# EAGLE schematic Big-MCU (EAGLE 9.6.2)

## Sheet 1 of 5: Board to Board Headers
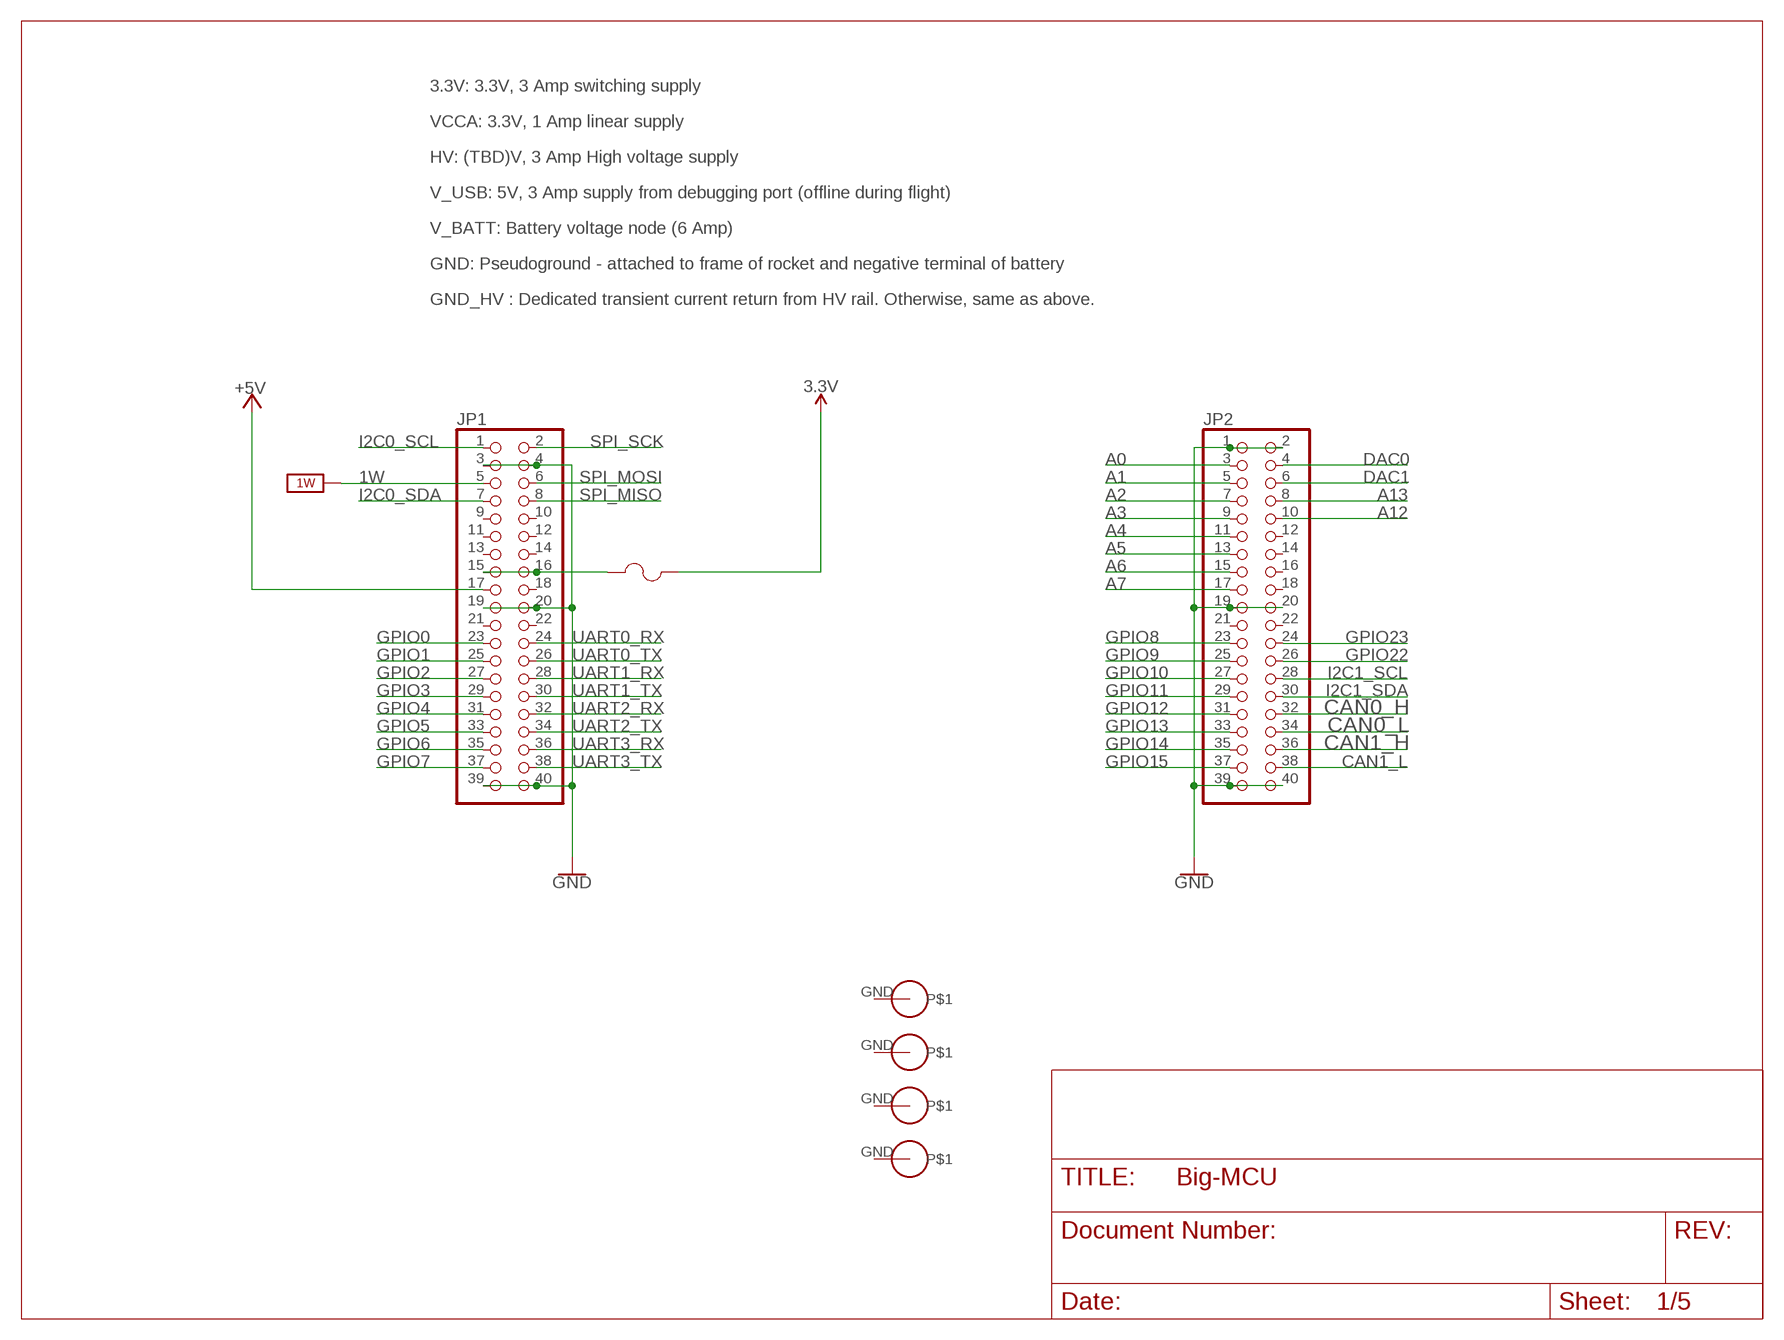
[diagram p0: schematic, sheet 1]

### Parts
$$U$1  PS/104-MOUNTING-HOLE  [PC/104-MOUNTING-HOLE]
F1  0603SFF150F/32-2  [FUS0603_TYCO]
JP1  PINHD-2X20  [2X20]
JP2  PINHD-2X20  [2X20]
U$1  PS/104-MOUNTING-HOLE  [PC/104-MOUNTING-HOLE]
U$2  PS/104-MOUNTING-HOLE  [PC/104-MOUNTING-HOLE]
U$3  PS/104-MOUNTING-HOLE  [PC/104-MOUNTING-HOLE]

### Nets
1W: JP1.5 ; supply symbol labelled 1W_SUP ; also sheet 3
3.3V [New Class]: F1.2 ; also sheet 2,4
+5V: JP1.17 ; also sheet 5
A0: JP2.3 ; also sheet 2
A1: JP2.5 ; also sheet 2
A2: JP2.7 ; also sheet 2
A3: JP2.9 ; also sheet 2
A4: JP2.11 ; also sheet 2
A5: JP2.13 ; also sheet 2
A6: JP2.15 ; also sheet 2
A7: JP2.17 ; also sheet 2
A12: JP2.10 ; also sheet 2
A13: JP2.8 ; also sheet 2
CAN0_H: JP2.32 ; also sheet 5
CAN0_L: JP2.34 ; also sheet 5
CAN1_H: JP2.36 ; also sheet 5
CAN1_L: JP2.38 ; also sheet 5
DAC0: JP2.4 ; also sheet 2
DAC1: JP2.6 ; also sheet 2
GND [New Class]: JP1.3 JP1.4 JP1.19 JP1.20 JP1.39 JP1.40 JP2.1 JP2.2 JP2.19 JP2.20 JP2.39 JP2.40 ; also sheet 2,3,4,5
GPIO0: JP1.23 ; also sheet 2
GPIO1: JP1.25 ; also sheet 2
GPIO2: JP1.27 ; also sheet 2
GPIO3: JP1.29 ; also sheet 2
GPIO4: JP1.31 ; also sheet 2
GPIO5: JP1.33 ; also sheet 2
GPIO6: JP1.35 ; also sheet 2
GPIO7: JP1.37 ; also sheet 2
GPIO8: JP2.23 ; also sheet 2
GPIO9: JP2.25 ; also sheet 2
GPIO10: JP2.27 ; also sheet 2
GPIO11: JP2.29 ; also sheet 2
GPIO12: JP2.31 ; also sheet 2
GPIO13: JP2.33 ; also sheet 2
GPIO14: JP2.35 ; also sheet 2
GPIO15: JP2.37 ; also sheet 2
GPIO22: JP2.26 ; also sheet 2
GPIO23: JP2.24 ; also sheet 2
I2C0_SCL: JP1.1 ; also sheet 2,3
I2C0_SDA: JP1.7 ; also sheet 2,3
I2C1_SCL: JP2.28 ; also sheet 2
I2C1_SDA: JP2.30 ; also sheet 2
N$3: F1.1 JP1.15 JP1.16
SPI_MISO: JP1.8 ; also sheet 2
SPI_MOSI: JP1.6 ; also sheet 4
SPI_SCK: JP1.2 ; also sheet 4
UART0_RX: JP1.24 ; also sheet 2
UART0_TX: JP1.26 ; also sheet 2
UART1_RX: JP1.28 ; also sheet 2
UART1_TX: JP1.30 ; also sheet 2
UART2_RX: JP1.32 ; also sheet 2
UART2_TX: JP1.34 ; also sheet 2
UART3_RX: JP1.36 ; also sheet 2
UART3_TX: JP1.38 ; also sheet 2
Unconnected: $$U$1.GND JP1.9 JP1.10 JP1.11 JP1.12 JP1.13 JP1.14 JP1.18 JP1.21 JP1.22 JP2.12 JP2.14 JP2.16 JP2.18 JP2.21 JP2.22 U$1.GND U$2.GND U$3.GND

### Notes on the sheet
- 3.3V: 3.3V, 3 Amp switching supply
- VCCA: 3.3V, 1 Amp linear supply
- HV: (TBD)V, 3 Amp High voltage supply
- V_USB: 5V, 3 Amp supply from debugging port (offline during flight)
- V_BATT: Battery voltage node (6 Amp)
- GND: Pseudoground - attached to frame of rocket and negative terminal of battery
- GND_HV : Dedicated transient current return from HV rail. Otherwise, same as above.

## Sheet 2 of 5: MCU
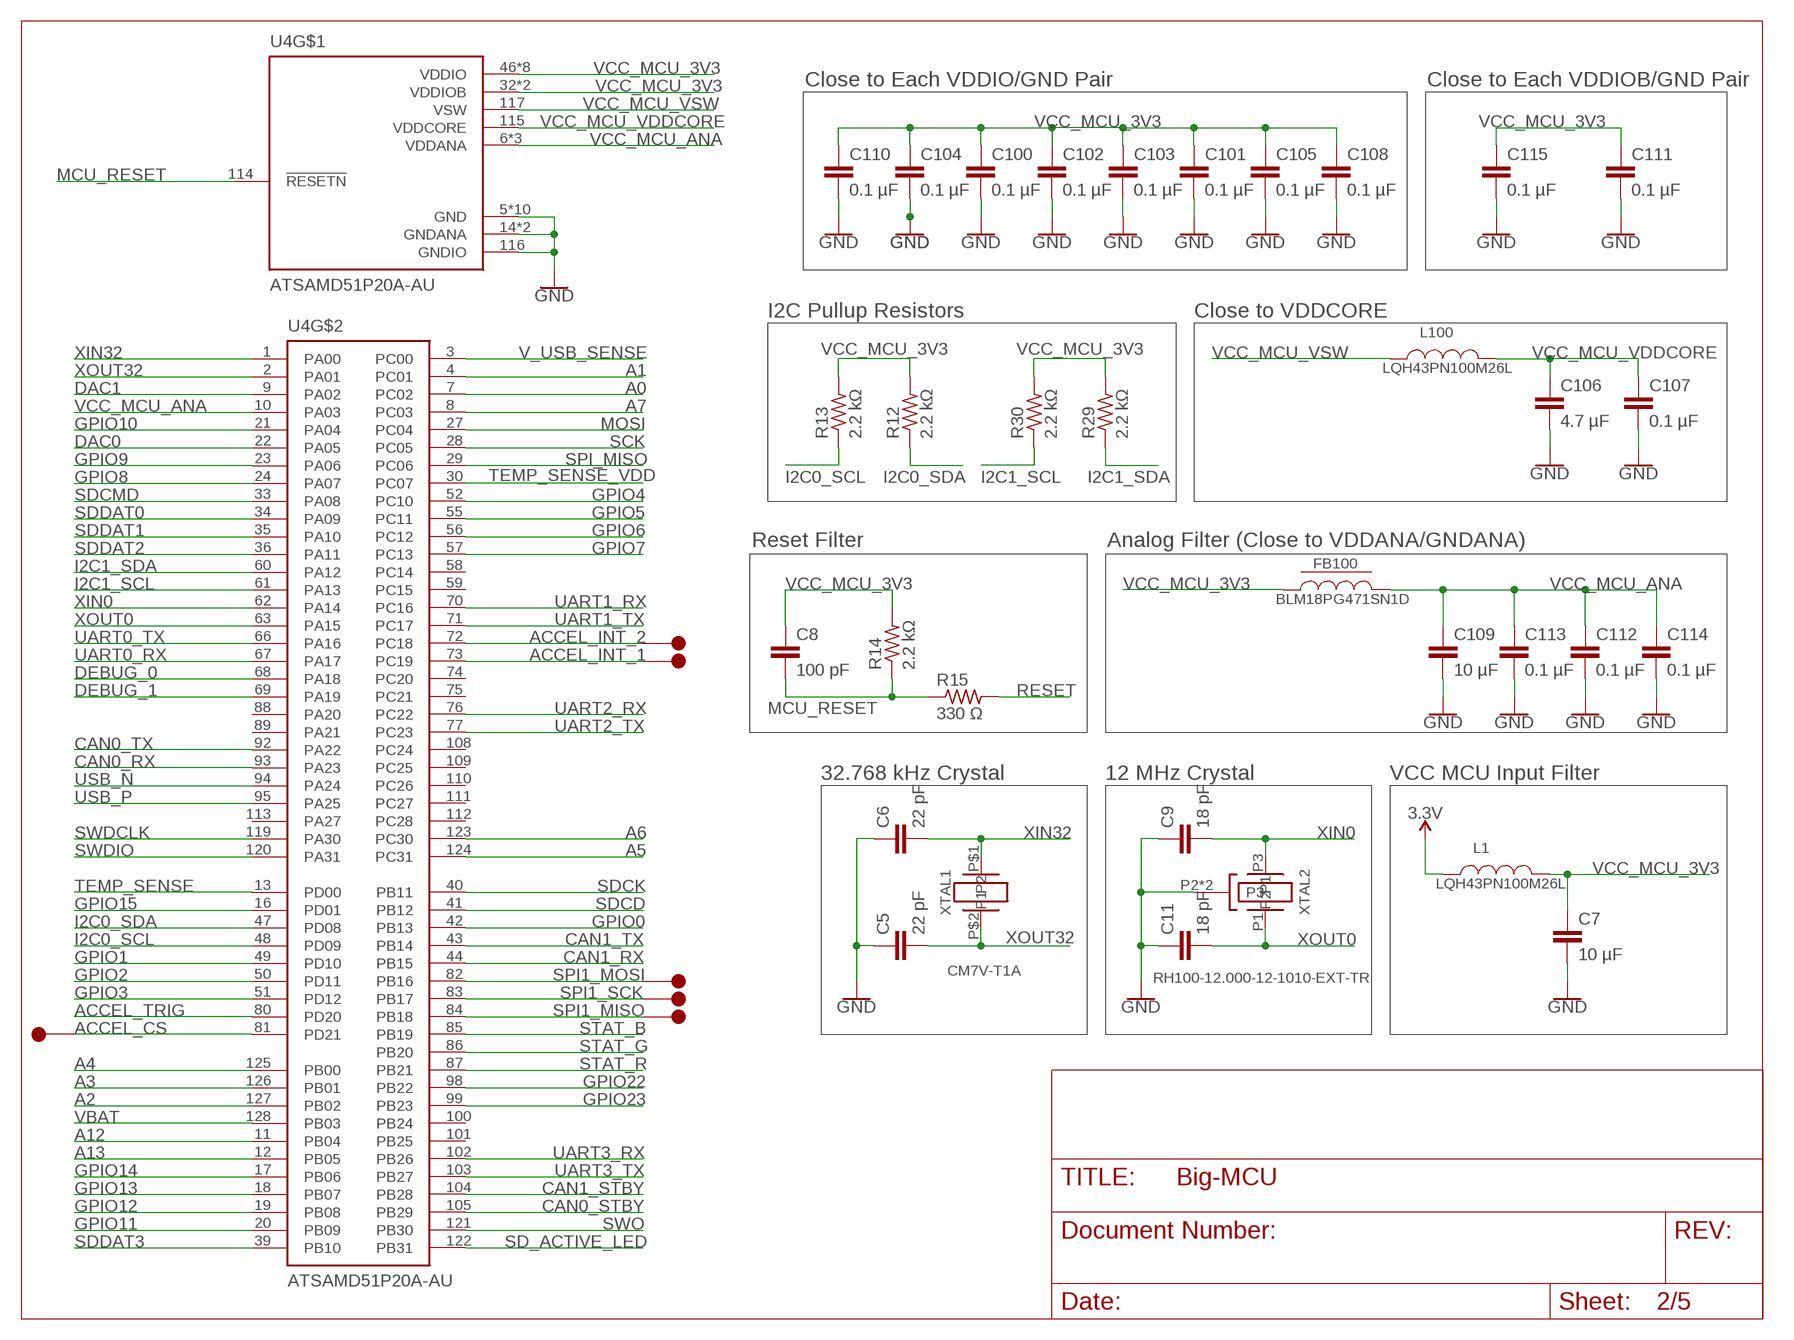
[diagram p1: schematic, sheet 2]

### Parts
C5  22 pF  C-EUC0805  [C0805]
C6  22 pF  C-EUC0805  [C0805]
C7  10 µF  C-EUC1206  [C1206]
C8  100 pF  C-EUC0805  [C0805]
C9  18 pF  C-EUC0805  [C0805]
C11  18 pF  C-EUC0805  [C0805]
C100  0.1 µF  C-EUC0805  [C0805]
C101  0.1 µF  C-EUC0805  [C0805]
C102  0.1 µF  C-EUC0805  [C0805]
C103  0.1 µF  C-EUC0805  [C0805]
C104  0.1 µF  C-EUC0805  [C0805]
C105  0.1 µF  C-EUC0805  [C0805]
C106  4.7 µF  C-EUC0805  [C0805]
C107  0.1 µF  C-EUC0805  [C0805]
C108  0.1 µF  C-EUC0805  [C0805]
C109  10 µF  C-EUC1206  [C1206]
C110  0.1 µF  C-EUC0805  [C0805]
C111  0.1 µF  C-EUC0805  [C0805]
C112  0.1 µF  C-EUC0805  [C0805]
C113  0.1 µF  C-EUC0805  [C0805]
C114  0.1 µF  C-EUC0805  [C0805]
C115  0.1 µF  C-EUC0805  [C0805]
FB100  BLM18PG471SN1D  [0603]
L1  LQH43PN100M26L  [LQH43PN100M26L]
L100  LQH43PN100M26L  [LQH43PN100M26L]
R12  2.2 kΩ  R-US_R0805  [R0805]
R13  2.2 kΩ  R-US_R0805  [R0805]
R14  2.2 kΩ  R-US_R0805  [R0805]
R15  330 Ω  R-US_R0805  [R0805]
R29  2.2 kΩ  R-US_R0805  [R0805]
R30  2.2 kΩ  R-US_R0805  [R0805]
TP11  5015  [KEYSTONE_5015]
TP12  5015  [KEYSTONE_5015]
TP13  5015  [KEYSTONE_5015]
TP14  5015  [KEYSTONE_5015]
TP15  5015  [KEYSTONE_5015]
TP16  5015  [KEYSTONE_5015]
U4  ATSAMD51P20A-AU  [QFP40P1600X1600X120-128N]
XTAL1  CM7V-T1A  CM7V-T1A-32.768KHZ-12.5PF-10PPM-TA-QC  [CM7V-T1A-32.768KHZ-12.5PF-10PPM-TA-QC]
XTAL2  RH100-12.000-12-1010-EXT-TR  [RH100-12.000-12-1010-EXT-TR]

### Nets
3.3V [New Class]: L1.1 ; also sheet 1,4
A0: U4.7(PC02) ; also sheet 1
A1: U4.4(PC01) ; also sheet 1
A2: U4.127(PB02) ; also sheet 1
A3: U4.126(PB01) ; also sheet 1
A4: U4.125(PB00) ; also sheet 1
A5: U4.124(PC31) ; also sheet 1
A6: U4.123(PC30) ; also sheet 1
A7: U4.8(PC03) ; also sheet 1
A12: U4.11(PB04) ; also sheet 1
A13: U4.12(PB05) ; also sheet 1
ACCEL_CS: TP15.1(TP) U4.81(PD21) ; also sheet 3
ACCEL_INT_1: TP11.1(TP) U4.73(PC19) ; also sheet 3
ACCEL_INT_2: TP13.1(TP) U4.72(PC18) ; also sheet 3
ACCEL_TRIG: U4.80(PD20) ; also sheet 3
CAN0_RX: U4.93(PA23) ; also sheet 5
CAN0_STBY: U4.105(PB29) ; also sheet 5
CAN0_TX: U4.92(PA22) ; also sheet 5
CAN1_RX: U4.44(PB15) ; also sheet 5
CAN1_STBY: U4.104(PB28) ; also sheet 5
CAN1_TX: U4.43(PB14) ; also sheet 5
DAC0: U4.22(PA05) ; also sheet 1
DAC1: U4.9(PA02) ; also sheet 1
DEBUG_0: U4.68(PA18) ; also sheet 3
DEBUG_1: U4.69(PA19) ; also sheet 3
GND [New Class]: C5.1 C6.1 C7.2 C9.1 C11.1 C100.2 C101.2 C102.2 C103.2 C104.2 C105.2 C106.2 C107.2 C108.2 C109.2 C110.2 C111.2 C112.2 C113.2 C114.2 C115.2 U4.5(GND) U4.14(GNDANA) U4.25(GNDANA) U4.31(GND) U4.38(GND) U4.45(GND) U4.53(GND) U4.64(GND) U4.78(GND) U4.90(GND) U4.96(GND) U4.106(GND) U4.116(GNDIO) XTAL2.P2(P3) XTAL2.P4(P3) ; also sheet 1,3,4,5
GPIO0: U4.42(PB13) ; also sheet 1
GPIO1: U4.49(PD10) ; also sheet 1
GPIO2: U4.50(PD11) ; also sheet 1
GPIO3: U4.51(PD12) ; also sheet 1
GPIO4: U4.52(PC10) ; also sheet 1
GPIO5: U4.55(PC11) ; also sheet 1
GPIO6: U4.56(PC12) ; also sheet 1
GPIO7: U4.57(PC13) ; also sheet 1
GPIO8: U4.24(PA07) ; also sheet 1
GPIO9: U4.23(PA06) ; also sheet 1
GPIO10: U4.21(PA04) ; also sheet 1
GPIO11: U4.20(PB09) ; also sheet 1
GPIO12: U4.19(PB08) ; also sheet 1
GPIO13: U4.18(PB07) ; also sheet 1
GPIO14: U4.17(PB06) ; also sheet 1
GPIO15: U4.16(PD01) ; also sheet 1
GPIO22: U4.98(PB22) ; also sheet 1
GPIO23: U4.99(PB23) ; also sheet 1
I2C0_SCL: R13.1 U4.48(PD09) ; also sheet 1,3
I2C0_SDA: R12.1 U4.47(PD08) ; also sheet 1,3
I2C1_SCL: R30.1 U4.61(PA13) ; also sheet 1
I2C1_SDA: R29.1 U4.60(PA12) ; also sheet 1
MCU_RESET: C8.2 R14.1 R15.1 U4.114(!RESETN)
MOSI: U4.27(PC04) ; also sheet 4
RESET: R15.2 ; also sheet 4
SCK: U4.28(PC05) ; also sheet 4
SD_ACTIVE_LED: U4.122(PB31) ; also sheet 3
SDCD: U4.41(PB12) ; also sheet 3
SDCK: U4.40(PB11) ; also sheet 3
SDCMD: U4.33(PA08) ; also sheet 3
SDDAT0: U4.34(PA09) ; also sheet 3
SDDAT1: U4.35(PA10) ; also sheet 3
SDDAT2: U4.36(PA11) ; also sheet 3
SDDAT3: U4.39(PB10) ; also sheet 3
SPI1_MISO: TP16.1(TP) U4.84(PB18) ; also sheet 3
SPI1_MOSI: TP12.1(TP) U4.82(PB16) ; also sheet 3
SPI1_SCK: TP14.1(TP) U4.83(PB17) ; also sheet 3
SPI_MISO: U4.29(PC06) ; also sheet 1
STAT_B: U4.85(PB19) ; also sheet 3
STAT_G: U4.86(PB20) ; also sheet 3
STAT_R: U4.87(PB21) ; also sheet 3
SWDCLK: U4.119(PA30) ; also sheet 4
SWDIO: U4.120(PA31) ; also sheet 4
SWO: U4.121(PB30) ; also sheet 4
TEMP_SENSE: U4.13(PD00) ; also sheet 3
TEMP_SENSE_VDD: U4.30(PC07) ; also sheet 3
UART0_RX: U4.67(PA17) ; also sheet 1
UART0_TX: U4.66(PA16) ; also sheet 1
UART1_RX: U4.70(PC16) ; also sheet 1
UART1_TX: U4.71(PC17) ; also sheet 1
UART2_RX: U4.76(PC22) ; also sheet 1
UART2_TX: U4.77(PC23) ; also sheet 1
UART3_RX: U4.102(PB26) ; also sheet 1
UART3_TX: U4.103(PB27) ; also sheet 1
USB_N: U4.94(PA24) ; also sheet 4
USB_P: U4.95(PA25) ; also sheet 4
V_USB_SENSE: U4.3(PC00) ; also sheet 4
VBAT: U4.128(PB03) ; also sheet 3
VCC_MCU_3V3 [New Class]: C7.1 C8.1 C100.1 C101.1 C102.1 C103.1 C104.1 C105.1 C108.1 C110.1 C111.1 C115.1 FB100.1 L1.2 R12.2 R13.2 R14.2 R29.2 R30.2 U4.32(VDDIOB) U4.37(VDDIOB) U4.46(VDDIO) U4.54(VDDIO) U4.65(VDDIO) U4.79(VDDIO) U4.91(VDDIO) U4.97(VDDIO) U4.107(VDDIO) U4.118(VDDIO) ; also sheet 3,4,5
VCC_MCU_ANA [New Class]: C109.1 C112.1 C113.1 C114.1 FB100.2 U4.6(VDDANA) U4.10(PA03) U4.15(VDDANA) U4.26(VDDANA)
VCC_MCU_VDDCORE [New Class]: C106.1 C107.1 L100.2 U4.115(VDDCORE)
VCC_MCU_VSW [New Class]: L100.1 U4.117(VSW)
XIN0: C9.2 U4.62(PA14) XTAL2.P3(P2)
XIN32: C6.2 U4.1(PA00) XTAL1.P$1(P1)
XOUT0: C11.2 U4.63(PA15) XTAL2.P1
XOUT32: C5.2 U4.2(PA01) XTAL1.P$2(P2)
Unconnected: U4.58(PC14) U4.59(PC15) U4.74(PC20) U4.75(PC21) U4.88(PA20) U4.89(PA21) U4.100(PB24) U4.101(PB25) U4.108(PC24) U4.109(PC25) U4.110(PC26) U4.111(PC27) U4.112(PC28) U4.113(PA27)

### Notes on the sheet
- Close to Each VDDIO/GND Pair | Close to Each VDDIOB/GND Pair
- I2C Pullup Resistors | Close to VDDCORE
- Reset Filter | Analog Filter (Close to VDDANA/GNDANA)
- 32.768 kHz Crystal | 12 MHz Crystal | VCC MCU Input Filter

## Sheet 3 of 5: Peripherals
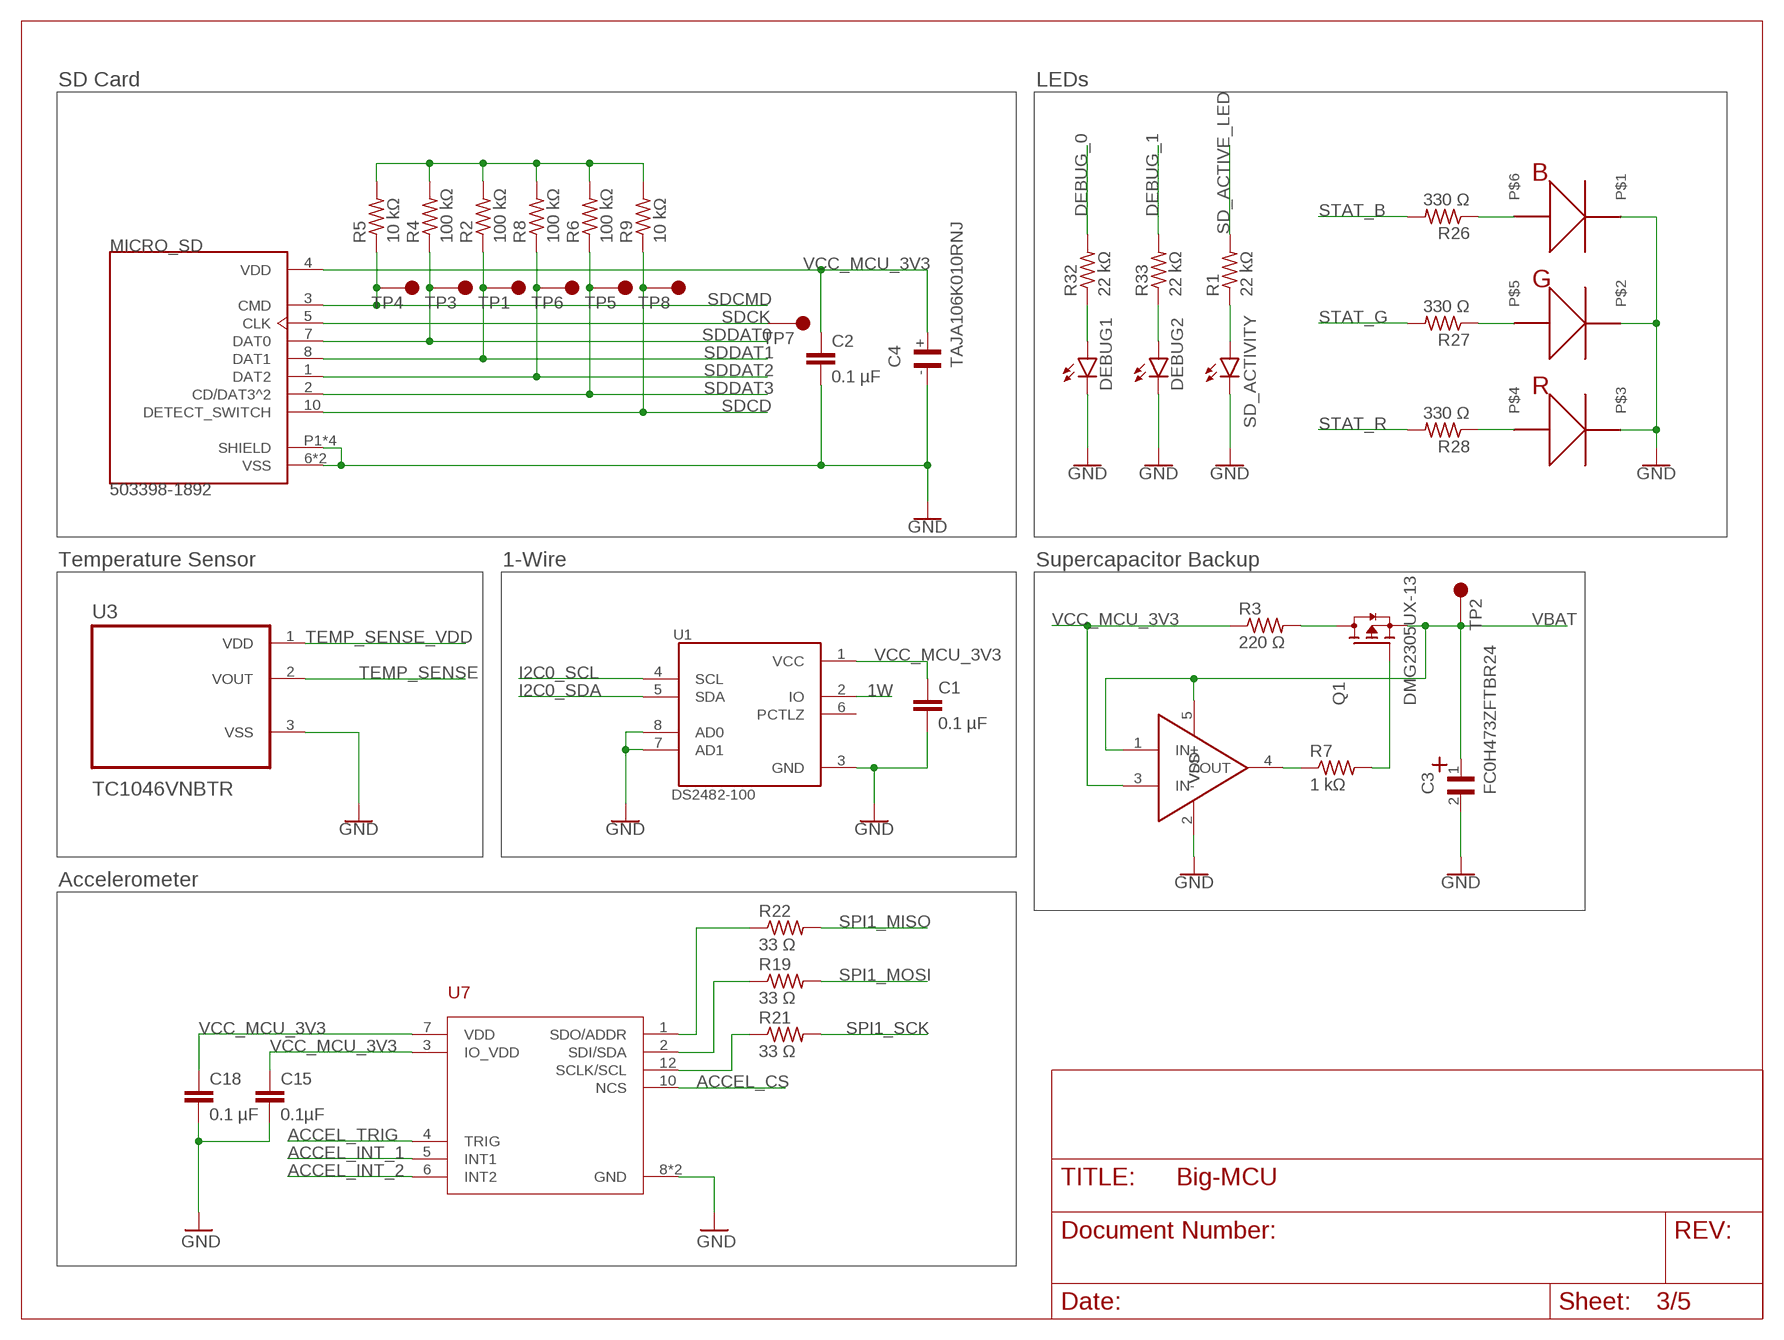
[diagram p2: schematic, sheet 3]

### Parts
C1  0.1 µF  C-EUC0805  [C0805]
C2  0.1 µF  C-EUC0805  [C0805]
C3  FC0H473ZFTBR24  [CAPAE1080X580N]
C4  TAJA106K010RNJ  [1206-POL]
C15  0.1µF  C-EUC0805  [C0805]
C18  0.1 µF  C-EUC0805  [C0805]
DEBUG1  LEDSML0805  [SML0805]
DEBUG2  LEDSML0805  [SML0805]
MICRO_SD  503398-1892  [MOLEX_503398-1892]
Q1  DMG2305UX-13  [SOT91P240X110-3N]
R1  22 kΩ  R-US_R0805  [R0805]
R2  100 kΩ  R-US_R0805  [R0805]
R3  220 Ω  R-US_R0805  [R0805]
R4  100 kΩ  R-US_R0805  [R0805]
R5  10 kΩ  R-US_R0805  [R0805]
R6  100 kΩ  R-US_R0805  [R0805]
R7  1 kΩ  R-US_R0805  [R0805]
R8  100 kΩ  R-US_R0805  [R0805]
R9  10 kΩ  R-US_R0805  [R0805]
R19  33 Ω  R-US_R0805  [R0805]
R21  33 Ω  R-US_R0805  [R0805]
R22  33 Ω  R-US_R0805  [R0805]
R26  330 Ω  R-US_R0805  [R0805]
R27  330 Ω  R-US_R0805  [R0805]
R28  330 Ω  R-US_R0805  [R0805]
R32  22 kΩ  R-US_R0805  [R0805]
R33  22 kΩ  R-US_R0805  [R0805]
SD_ACTIVITY  LEDSML0805  [SML0805]
STATUS  MSL0402RGB  [MSL0402RGB]
TP1  5015  [KEYSTONE_5015]
TP2  5015  [KEYSTONE_5015]
TP3  5015  [KEYSTONE_5015]
TP4  5015  [KEYSTONE_5015]
TP5  5015  [KEYSTONE_5015]
TP6  5015  [KEYSTONE_5015]
TP7  5015  [KEYSTONE_5015]
TP8  5015  [KEYSTONE_5015]
U1  DS2482-100  [SOIC8]
U2  BU7265SG-TR  [SOT95P285X145-5N]
U3  TC1046VNBTR  [SOT95P237X112-3N]
U7  KX134-1211  [KX134-1211]

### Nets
1W: U1.2(IO) ; also sheet 1
ACCEL_CS: U7.10(NCS) ; also sheet 2
ACCEL_INT_1: U7.5(INT1) ; also sheet 2
ACCEL_INT_2: U7.6(INT2) ; also sheet 2
ACCEL_TRIG: U7.4(TRIG) ; also sheet 2
DEBUG_0: R32.2 ; also sheet 2
DEBUG_1: R33.2 ; also sheet 2
GND [New Class]: C1.2 C2.2 C3.2 C4.- C15.2 C18.2 DEBUG1.C DEBUG2.C MICRO_SD.6(VSS) MICRO_SD.9(VSS) MICRO_SD.P1(SHIELD) MICRO_SD.P2(SHIELD) MICRO_SD.P3(SHIELD) MICRO_SD.P4(SHIELD) SD_ACTIVITY.C STATUS.P1 STATUS.P2 STATUS.P3 U1.3(GND) U1.7(AD1) U1.8(AD0) U2.2(VSS) U3.3(VSS) U7.8(GND) U7.9(GND) ; also sheet 1,2,4,5
I2C0_SCL: U1.4(SCL) ; also sheet 1,2
I2C0_SDA: U1.5(SDA) ; also sheet 1,2
N$1: R1.1 SD_ACTIVITY.A
N$4: DEBUG2.A R33.1
N$5: R26.1 STATUS.P6
N$7: DEBUG1.A R32.1
N$8: R27.1 STATUS.P5
N$9: R28.1 STATUS.P4
N$10: R21.1 U7.12(SCLK/SCL)
N$11: R19.1 U7.2(SDI/SDA)
N$13: R22.1 U7.1(SDO/ADDR)
N$14: R7.1 U2.4(OUT)
N$16: Q1.1(G) R7.2
N$18: Q1.3(D) R3.2
SD_ACTIVE_LED: R1.2 ; also sheet 2
SDCD: MICRO_SD.10(DETECT_SWITCH) R9.1 TP8.1(TP) ; also sheet 2
SDCK: MICRO_SD.5(CLK) TP7.1(TP) ; also sheet 2
SDCMD: MICRO_SD.3(CMD) R5.1 TP4.1(TP) ; also sheet 2
SDDAT0: MICRO_SD.7(DAT0) R4.1 TP3.1(TP) ; also sheet 2
SDDAT1: MICRO_SD.8(DAT1) R2.1 TP1.1(TP) ; also sheet 2
SDDAT2: MICRO_SD.1(DAT2) R8.1 TP6.1(TP) ; also sheet 2
SDDAT3: MICRO_SD.2(CD/DAT3^2) R6.1 TP5.1(TP) ; also sheet 2
SPI1_MISO: R22.2 ; also sheet 2
SPI1_MOSI: R19.2 ; also sheet 2
SPI1_SCK: R21.2 ; also sheet 2
STAT_B: R26.2 ; also sheet 2
STAT_G: R27.2 ; also sheet 2
STAT_R: R28.2 ; also sheet 2
TEMP_SENSE: U3.2(VOUT) ; also sheet 2
TEMP_SENSE_VDD: U3.1(VDD) ; also sheet 2
VBAT: C3.1 Q1.2(S) TP2.1(TP) U2.1(IN+) U2.5(VDD) ; also sheet 2
VCC_MCU_3V3 [New Class]: C1.1 C2.1 C4.+ C15.1 C18.1 MICRO_SD.4(VDD) R2.2 R3.1 R4.2 R5.2 R6.2 R8.2 R9.2 U1.1(VCC) U2.3(IN-) U7.3(IO_VDD) U7.7(VDD) ; also sheet 2,4,5
Unconnected: U1.6(PCTLZ)

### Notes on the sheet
- SD Card | LEDs
- Temperature Sensor | 1-Wire | Supercapacitor Backup
- Accelerometer

## Sheet 4 of 5: Connector and Series Resitors
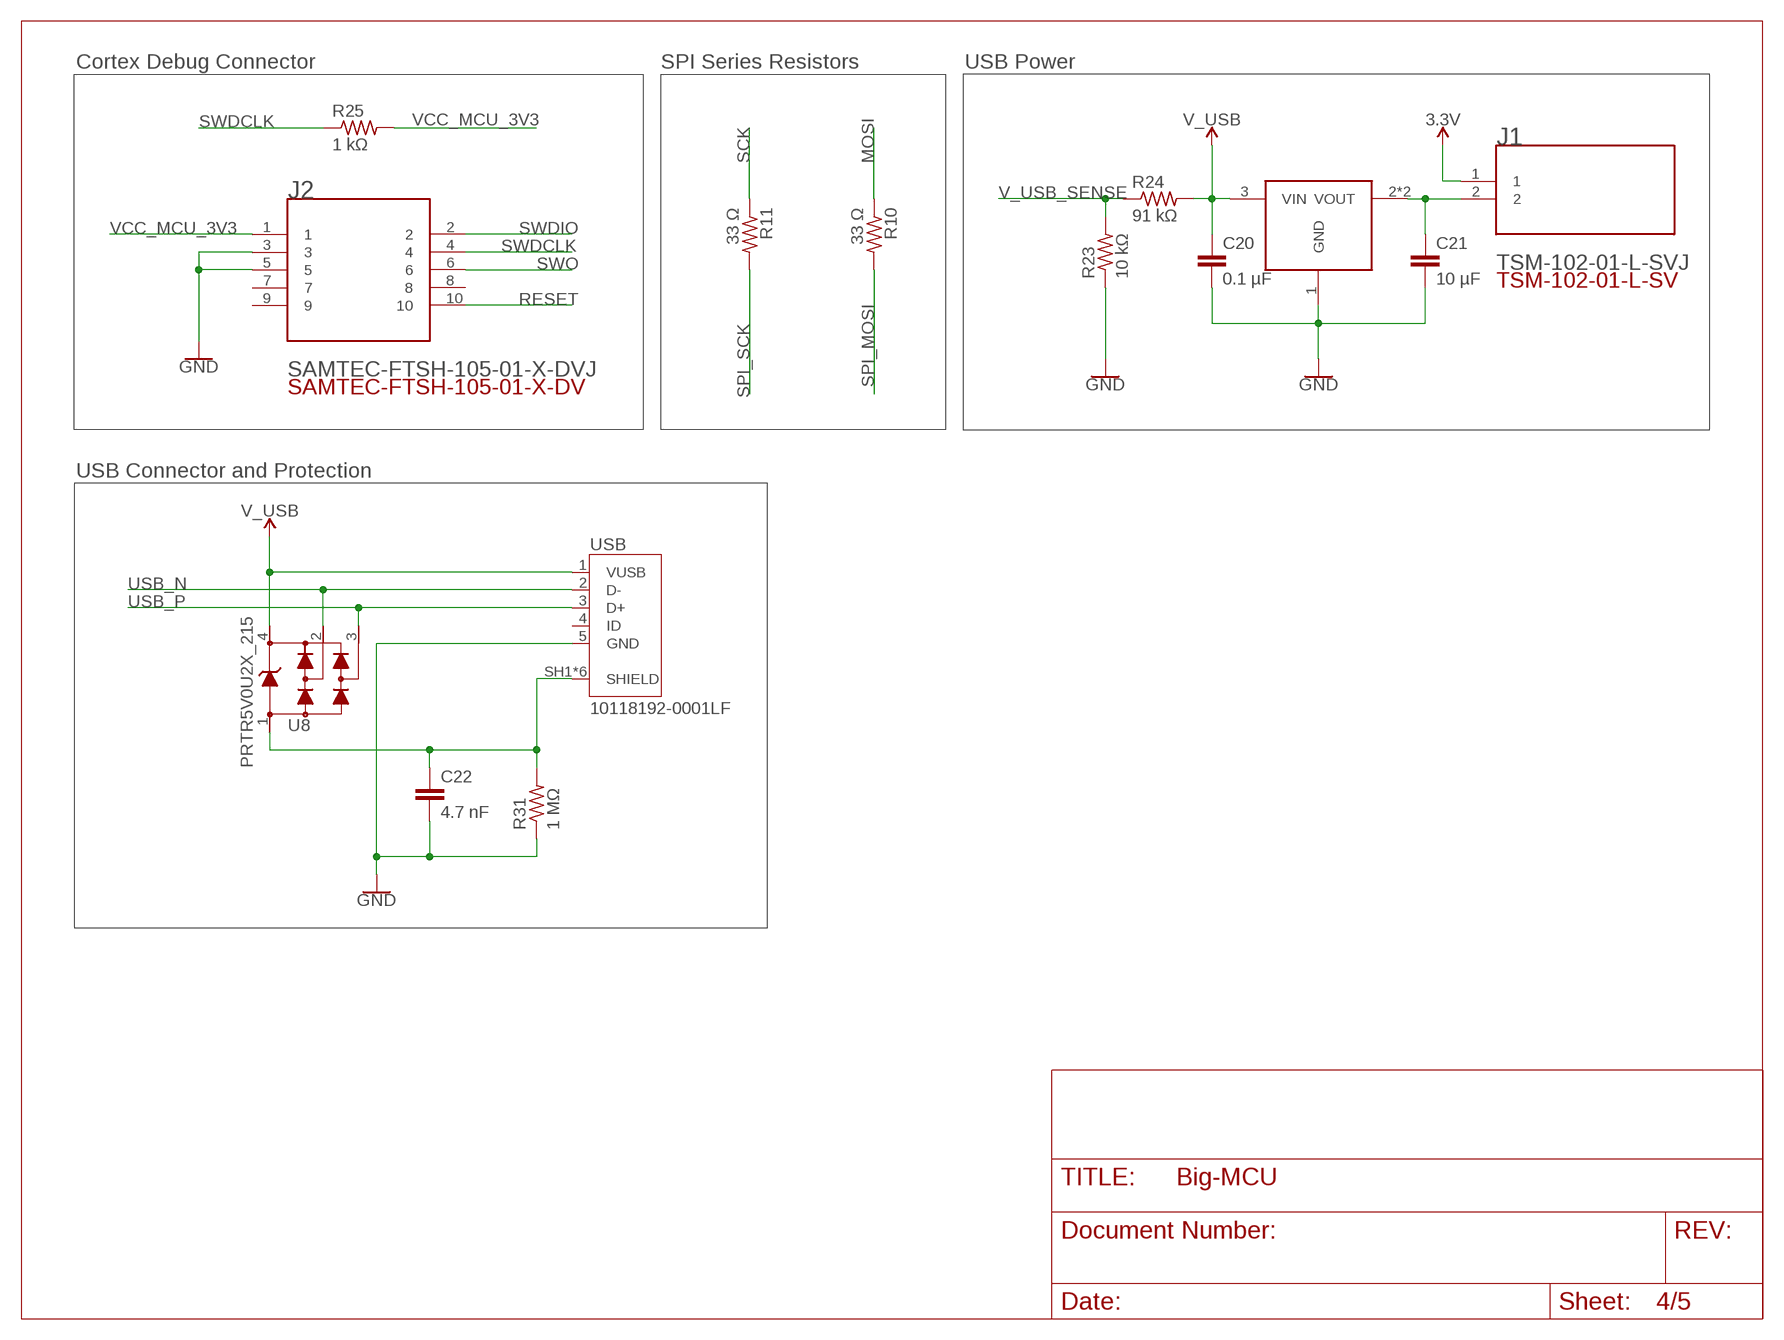
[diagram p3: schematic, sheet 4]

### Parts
C20  0.1 µF  C-EUC0805  [C0805]
C21  10 µF  C-EUC1206  [C1206]
C22  4.7 nF  C-EUC0805  [C0805]
J1  TSM-102-01-L-SVJ  [TSM-102-01-L-SV]
J2  SAMTEC-FTSH-105-01-X-DVJ  [SAMTEC-FTSH-105-01-X-DV]
R10  33 Ω  R-US_R0805  [R0805]
R11  33 Ω  R-US_R0805  [R0805]
R23  10 kΩ  R-US_R0805  [R0805]
R24  91 kΩ  R-US_R0805  [R0805]
R25  1 kΩ  R-US_R0805  [R0805]
R31  1 MΩ  R-US_R0805  [R0805]
U8  PRTR5V0U2X_215  [SOT143B]
U9  LDL1117S33R  [SOT223]
USB  10118192-0001LF  [10118192-0001LF]

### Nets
3.3V [New Class]: J1.1 ; also sheet 1,2
GND [New Class]: C20.2 C21.2 C22.2 J2.3 J2.5 R23.1 R31.1 U9.1(GND) USB.5(GND) ; also sheet 1,2,3,5
MOSI: R10.1 ; also sheet 2
N$2: C22.1 R31.2 U8.1 USB.SH1(SHIELD) USB.SH2(SHIELD) USB.SH3(SHIELD) USB.SH4(SHIELD) USB.SH5(SHIELD) USB.SH6(SHIELD)
N$6: C21.1 J1.2 U9.2(VOUT) U9.4(VOUT)
RESET: J2.10 ; also sheet 2
SCK: R11.1 ; also sheet 2
SPI_MOSI: R10.2 ; also sheet 1
SPI_SCK: R11.2 ; also sheet 1
SWDCLK: J2.4 R25.1 ; also sheet 2
SWDIO: J2.2 ; also sheet 2
SWO: J2.6 ; also sheet 2
USB_N: U8.2 USB.2(D-) ; also sheet 2
USB_P: U8.3 USB.3(D+) ; also sheet 2
V_USB [New Class]: C20.1 R24.2 U8.4 U9.3(VIN) USB.1(VUSB)
V_USB_SENSE: R23.2 R24.1 ; also sheet 2
VCC_MCU_3V3 [New Class]: J2.1 R25.2 ; also sheet 2,3,5
Unconnected: J2.7 J2.8 J2.9 USB.4(ID)

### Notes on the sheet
- Cortex Debug Connector | SPI Series Resistors | USB Power
- USB Connector and Protection

## Sheet 5 of 5: CAN
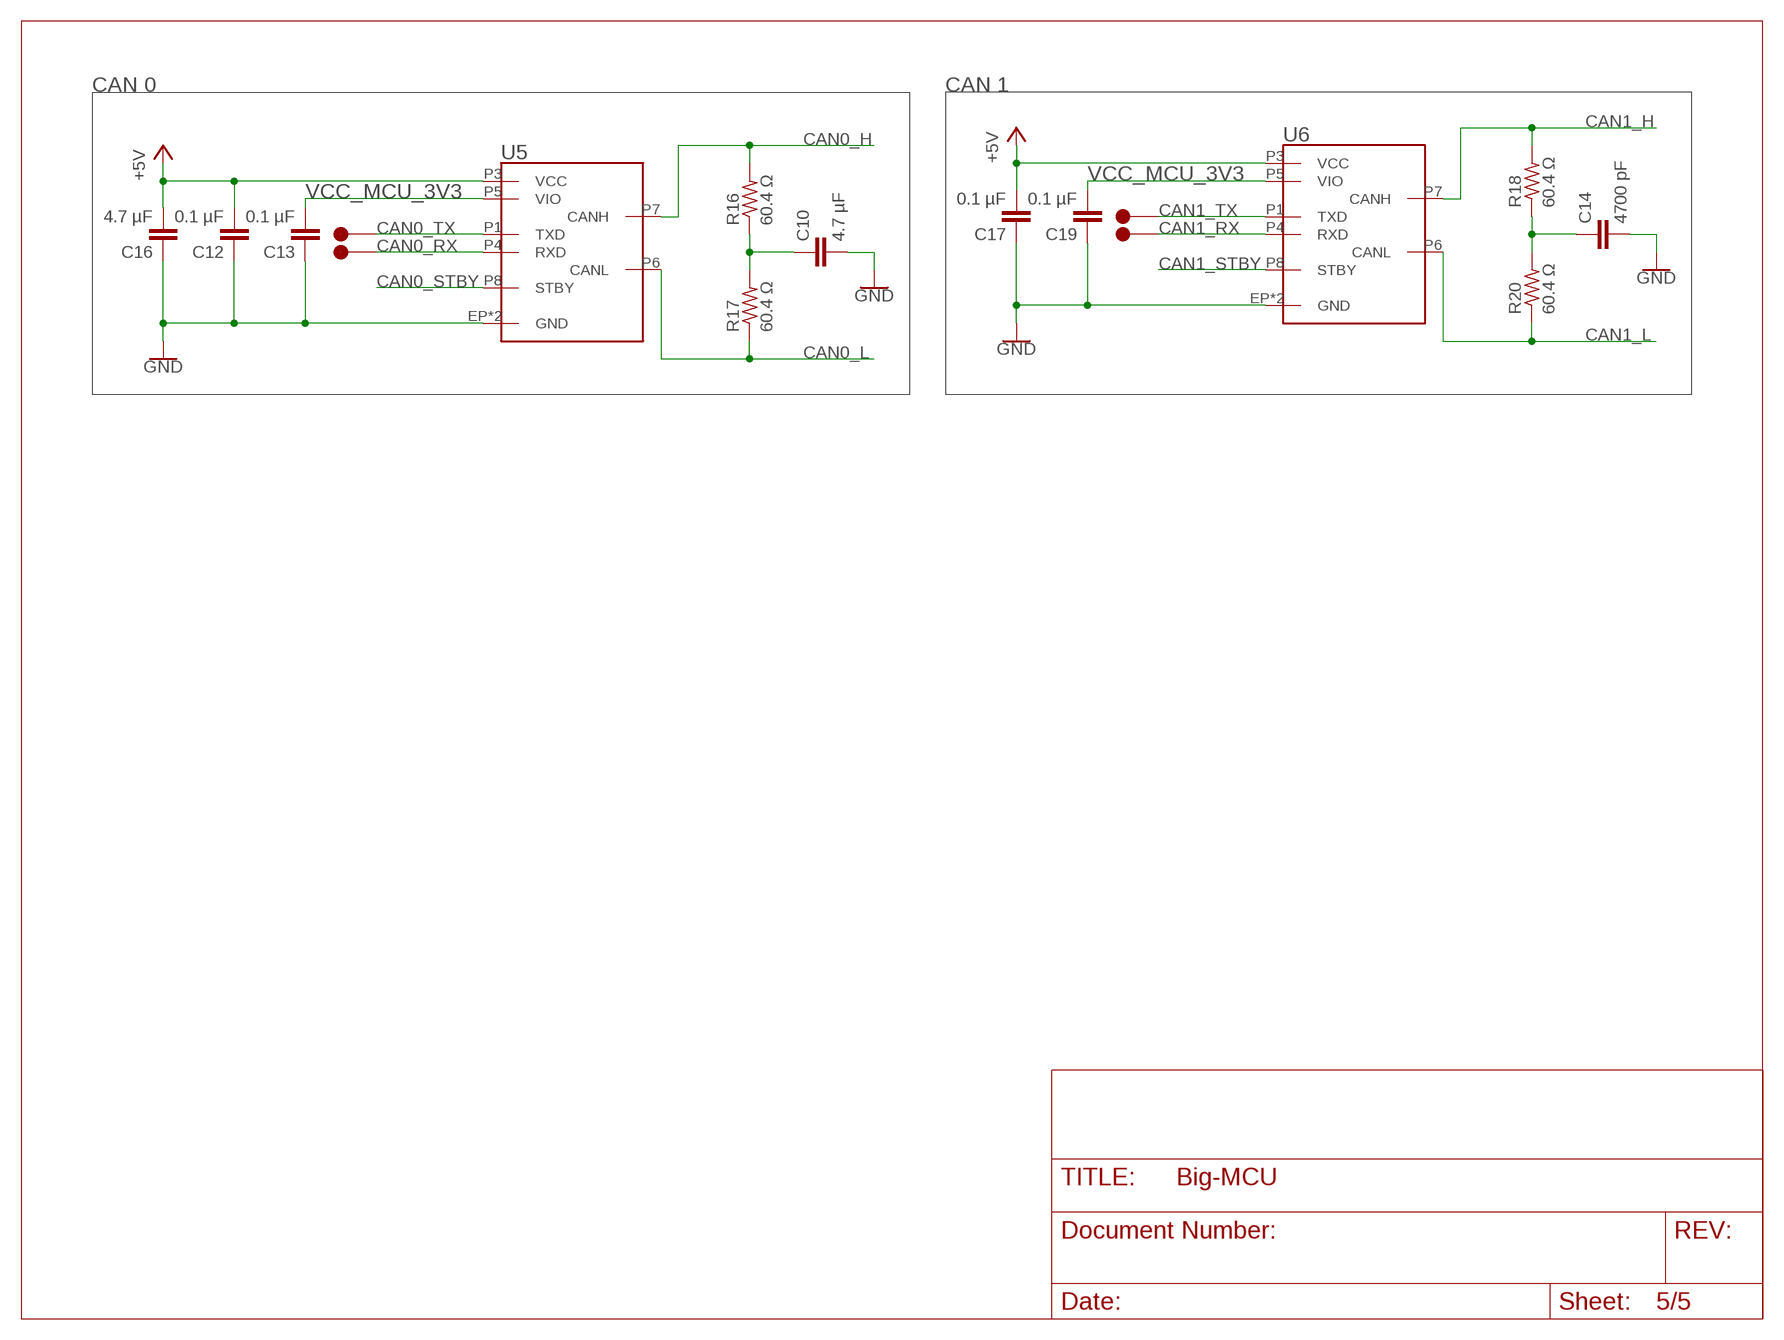
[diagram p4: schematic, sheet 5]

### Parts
C10  4.7 µF  C-EUC0805  [C0805]
C12  0.1 µF  C-EUC0805  [C0805]
C13  0.1 µF  C-EUC0805  [C0805]
C14  4700 pF  C-EUC0805  [C0805]
C16  4.7 µF  C-EUC0805  [C0805]
C17  0.1 µF  C-EUC0805  [C0805]
C19  0.1 µF  C-EUC0805  [C0805]
R16  60.4 Ω  R-US_R1206  [R1206]
R17  60.4 Ω  R-US_R1206  [R1206]
R18  60.4 Ω  R-US_R1206  [R1206]
R20  60.4 Ω  R-US_R1206  [R1206]
TP17  5015  [KEYSTONE_5015]
TP18  5015  [KEYSTONE_5015]
TP19  5015  [KEYSTONE_5015]
TP20  5015  [KEYSTONE_5015]
U5  ATA6561  [VDFN8]
U6  ATA6561  [VDFN8]

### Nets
+5V: C12.2 C16.2 C17.2 U5.P3(VCC) U6.P3(VCC) ; also sheet 1
CAN0_H: R16.2 U5.P7(CANH) ; also sheet 1
CAN0_L: R17.1 U5.P6(CANL) ; also sheet 1
CAN0_RX: TP17.1(TP) U5.P4(RXD) ; also sheet 2
CAN0_STBY: U5.P8(STBY) ; also sheet 2
CAN0_TX: TP18.1(TP) U5.P1(TXD) ; also sheet 2
CAN1_H: R18.2 U6.P7(CANH) ; also sheet 1
CAN1_L: R20.1 U6.P6(CANL) ; also sheet 1
CAN1_RX: TP20.1(TP) U6.P4(RXD) ; also sheet 2
CAN1_STBY: U6.P8(STBY) ; also sheet 2
CAN1_TX: TP19.1(TP) U6.P1(TXD) ; also sheet 2
GND [New Class]: C10.2 C12.1 C13.1 C14.2 C16.1 C17.1 C19.1 U5.EP(GND) U5.P2(GND) U6.EP(GND) U6.P2(GND) ; also sheet 1,2,3,4
N$12: C10.1 R16.1 R17.2
N$15: C14.1 R18.1 R20.2
VCC_MCU_3V3 [New Class]: C13.2 C19.2 U5.P5(VIO) U6.P5(VIO) ; also sheet 2,3,4

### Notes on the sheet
- CAN 0 | CAN 1

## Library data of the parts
$$U$1 U$1-U$3 = CU inSpace 2019 Parts:PS/104-MOUNTING-HOLE: Mounting hole for PC/104 board.
C1 C2 C5-C22 C100-C115 = rcl:C-EU: CAPACITOR, European symbol; SPICEPREFIX: C
C3 = MCU Board:FC0H473ZFTBR24
C4 = MCU Board:TAJA106K010RNJ
DEBUG1 DEBUG2 SD_ACTIVITY = led:LED: LED
F1 = CU inSpace 2019 Parts:0603SFF150F/32-2; MANUFACTURER_PART_NUMBER: 0603SFF150F322; VENDOR: Littelfuse Inc
FB100 = MCU Board:BLM18PG471SN1D
J1 = MCU Board:TSM-102-01-L-SV; DESCRIPTION: Connector Header Surface Mount 2 position 0.100 (2.54mm); DIGI-KEY_PART_NUMBER: SAM14923TR-ND; MF: Samtec; MP: TSM-102-01-L-SV; PACKAGE: None; TOBY_UK-PURCHASE-URL: https://snapeda.com/shop?store=Toby+UK&id=2748087
J2 = MCU Board:SAMTEC-FTSH-105-01-X-DV
JP1 JP2 = pinhead:PINHD-2X20: PIN HEADER
L1 L100 = MCU Board:LQH43PN100M26L
MICRO_SD = CUINSPACE_Managed:503398-1892
Q1 = MCU Board:DMG2305UX-13: DMG2305UX Series 20 V 65 Ohms P-Ch Enhancement Mode Mosfet - SOT-23-3 Check prices; AVAILABILITY: Good; DESCRIPTION: Trans MOSFET P-CH 20V 4.2A 3-Pin SOT-23 T/R; MF: Diodes Zetex; MP: DMG2305UX-13; PACKAGE: None; PRICE: None; PURCHASE-URL: https://pricing.snapeda.com/search/part/DMG2305UX-13/?ref=eda
R1-R33 = rcl:R-US_: RESISTOR, American symbol; SPICEPREFIX: R
STATUS = MCU Board:MSL0402RGB
TP1-TP8 TP11-TP20 = MCU Board:5015: Test Point; Black; Surface Mount; Wire Leaded; Polycarbonate; 0.04 in.; AVAILABILITY: Unavailable; DESCRIPTION: 2.2µH Shielded Wirewound Inductor 4A 52mOhm Max Nonstandard; MF: Keystone Electronics; MOUSER-PURCHASE-URL: https://snapeda.com/shop?store=Mouser&id=48459; MP: 5015; PACKAGE: Keystone Electronics; PRICE: None
U1 = MCU Board:DS2482-100
U2 = MCU Board:BU7265SG-TR
U3 = MCU Board:TC1046VNBTR: Buy Part; ARROW_ELECTRONICS-PURCHASE-URL: https://snapeda.com/shop?store=Arrow+Electronics&id=234729; AVAILABILITY: Good; DESCRIPTION: Temperature Sensor Analog, Local -40°C ~ 125°C 6.25mV/°C SOT-23-3; DIGIKEY-PURCHASE-URL: https://snapeda.com/shop?store=DigiKey&id=234729; MF: Microchip; MOUSER-PURCHASE-URL: https://snapeda.com/shop?store=Mouser&id=234729; MP: TC1046VNBTR; PACKAGE: SOT-23 Microchip; PRICE: None
U4 = MCU Board:ATSAMD51P20A-AU: SAMD51 Series 1 MB Flash 256 kB RAM 32-Bit SMT Microcontroller - TQFP-128; AVAILABILITY: Unavailable; DESCRIPTION: ARM® Cortex®-M4F SAM D51 Microcontroller IC 32-Bit 120MHz 1MB (1M x 8) FLASH 128-TQFP (14x14); MF: Microchip; MP: ATSAMD51P20A-AU; PACKAGE: TQFP-128 Microchip; PRICE: None
U5 U6 = MCU Board:ATA6561
U7 = MCU Board:KX134-1211
U8 = MCU Board:PRTR5V0U2X_215
U9 = MCU Board:LDL1117S33R
USB = MCU Board:10118192-0001LF
XTAL1 = MCU Board:CM7V-T1A-32.768KHZ-12.5PF-10PPM-TA-QC
XTAL2 = MCU Board:RH100-12.000-12-1010-EXT-TR

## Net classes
2 diff pairs: width 0.254 mm

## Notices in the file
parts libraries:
SparkFun-PowerSymbols: Licensing: Creative Commons ShareAlike 4.0 International - https://creativecommons.org/licenses/by-sa/4.0
